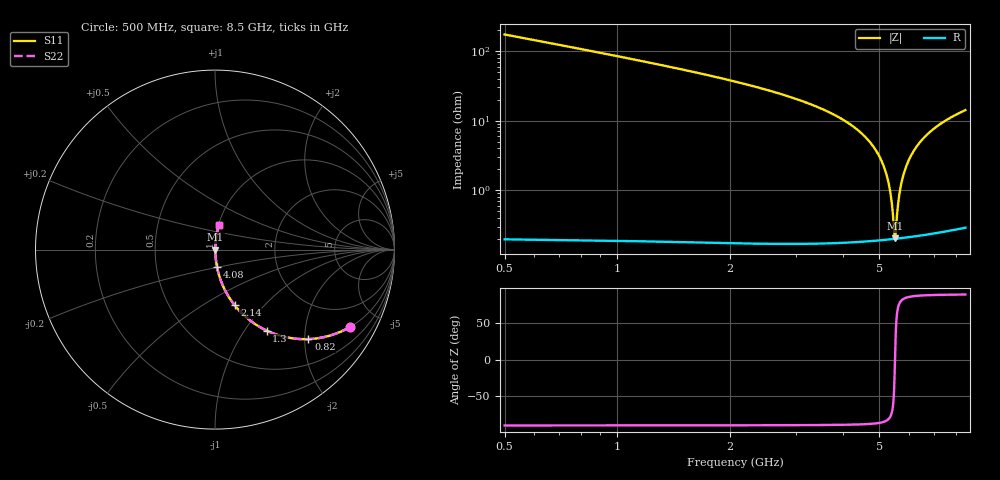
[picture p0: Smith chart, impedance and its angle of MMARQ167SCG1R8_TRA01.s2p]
! MMARQ167SCG1R8_TRA01  S-PARAMETER MODEL  ( General Type )
! Model Generated by TAIYO YUDEN Corporation (http://www.ty-top.com)
! Version 1.0
! TAIYO YUDEN Control No. 150305
! Copyright(c) 2015 TAIYO YUDEN CO.,LTD. All Rights Reserved.
! Product Description (link to TY-COMPAS)
! https://ds.yuden.co.jp/TYCOMPAS/or/detail?pn=MMARQ167SCG1R8BTRA01&u=M
! Products Name : Multilayer Ceramic Capacitors
! Characteristics :
!  Capacitance : 1.8 pF , Rated Voltage : 250V , TCC : CG / C0G
!  Case Size : 1.6 x 0.8 / 0.063 x 0.031 [mm/inch] , Thickness : 0.7 / 0.028 [mm/inch]
!  (Conditions: Temperature = 25 degC , DC Bias Current/Voltage = 0A / 0V)
! External Node Assignments :
!  1  o---| |---o  2
! GND o---------o GND
! Frequency Range : 500MHz  -  8.5GHz  [ 401 STEP ]
# MHz S RI R 50
! Freq[MHz].  S11 Real  S11 Imag  S21 Real  S21 Imag  S12 Real  S12 Imag  S22 Real  S22 Imag
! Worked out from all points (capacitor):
!   401 points, 500 MHz to 8.5 GHz, reference 50 ohm
!   read as one part in series: C = 1.82 pF near 540 MHz
!   lowest |Z| = 203 mohm at 5.52 GHz (marker M1)
!   series resonance near 5.514 GHz, so ESL is about 460 pH
!   S11 on the Smith chart (normalised r, x): 500 MHz: 1.00, -3.47; 820 MHz: 1.00, -2.08; 1.3 GHz: 1.00, -1.27; 2.14 GHz: 1.00, -0.69; 4.08 GHz: 1.00, -0.19; 8.5 GHz: 1.01, +0.28
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500  0.75 -0.4325  0.25 0.4325  0.25 0.4325  0.75 -0.4325
820  0.5206 -0.4987  0.4794 0.4987  0.4794 0.4987  0.5206 -0.4987
1300  0.2879 -0.4513  0.7121 0.4513  0.7121 0.4513  0.2879 -0.4513
1840  0.1523 -0.3573  0.8477 0.3573  0.8477 0.3573  0.1523 -0.3573
2140  0.1087 -0.3088  0.8913 0.3088  0.8913 0.3088  0.1087 -0.3088
3180  0.0341 -0.177  0.9659 0.177  0.9659 0.177  0.0341 -0.177
4080  0.011 -0.0958  0.989 0.0958  0.989 0.0958  0.011 -0.0958
4500  0.00598 -0.0644  0.994 0.0644  0.994 0.0644  0.00598 -0.0644
4920  0.00318 -0.036  0.9968 0.036  0.9968 0.036  0.00318 -0.036
5200  0.00227 -0.0185  0.9977 0.0185  0.9977 0.0185  0.00227 -0.0185
5360  0.00204 -0.00894  0.998 0.00894  0.998 0.00894  0.00204 -0.00894
5420  0.002 -0.00542  0.998 0.00542  0.998 0.00542  0.002 -0.00542
5480  0.00199 -0.00194  0.998 0.00194  0.998 0.00194  0.00199 -0.00194
5520  0.002 0.000361  0.998 -0.000361  0.998 -0.000361  0.002 0.000361
5540  0.002 0.0015  0.998 -0.0015  0.998 -0.0015  0.002 0.0015
5660  0.0021 0.00828  0.9979 -0.00828  0.9979 -0.00828  0.0021 0.00828
5740  0.00221 0.0127  0.9978 -0.0127  0.9978 -0.0127  0.00221 0.0127
5840  0.0024 0.0182  0.9976 -0.0182  0.9976 -0.0182  0.0024 0.0182
6060  0.00302 0.0299  0.997 -0.0299  0.997 -0.0299  0.00302 0.0299
6340  0.00415 0.0442  0.9958 -0.0442  0.9958 -0.0442  0.00415 0.0442
7180  0.00952 0.0838  0.9905 -0.0838  0.9905 -0.0838  0.00952 0.0838
8500  0.0224 0.1381  0.9776 -0.1381  0.9776 -0.1381  0.0224 0.1381
